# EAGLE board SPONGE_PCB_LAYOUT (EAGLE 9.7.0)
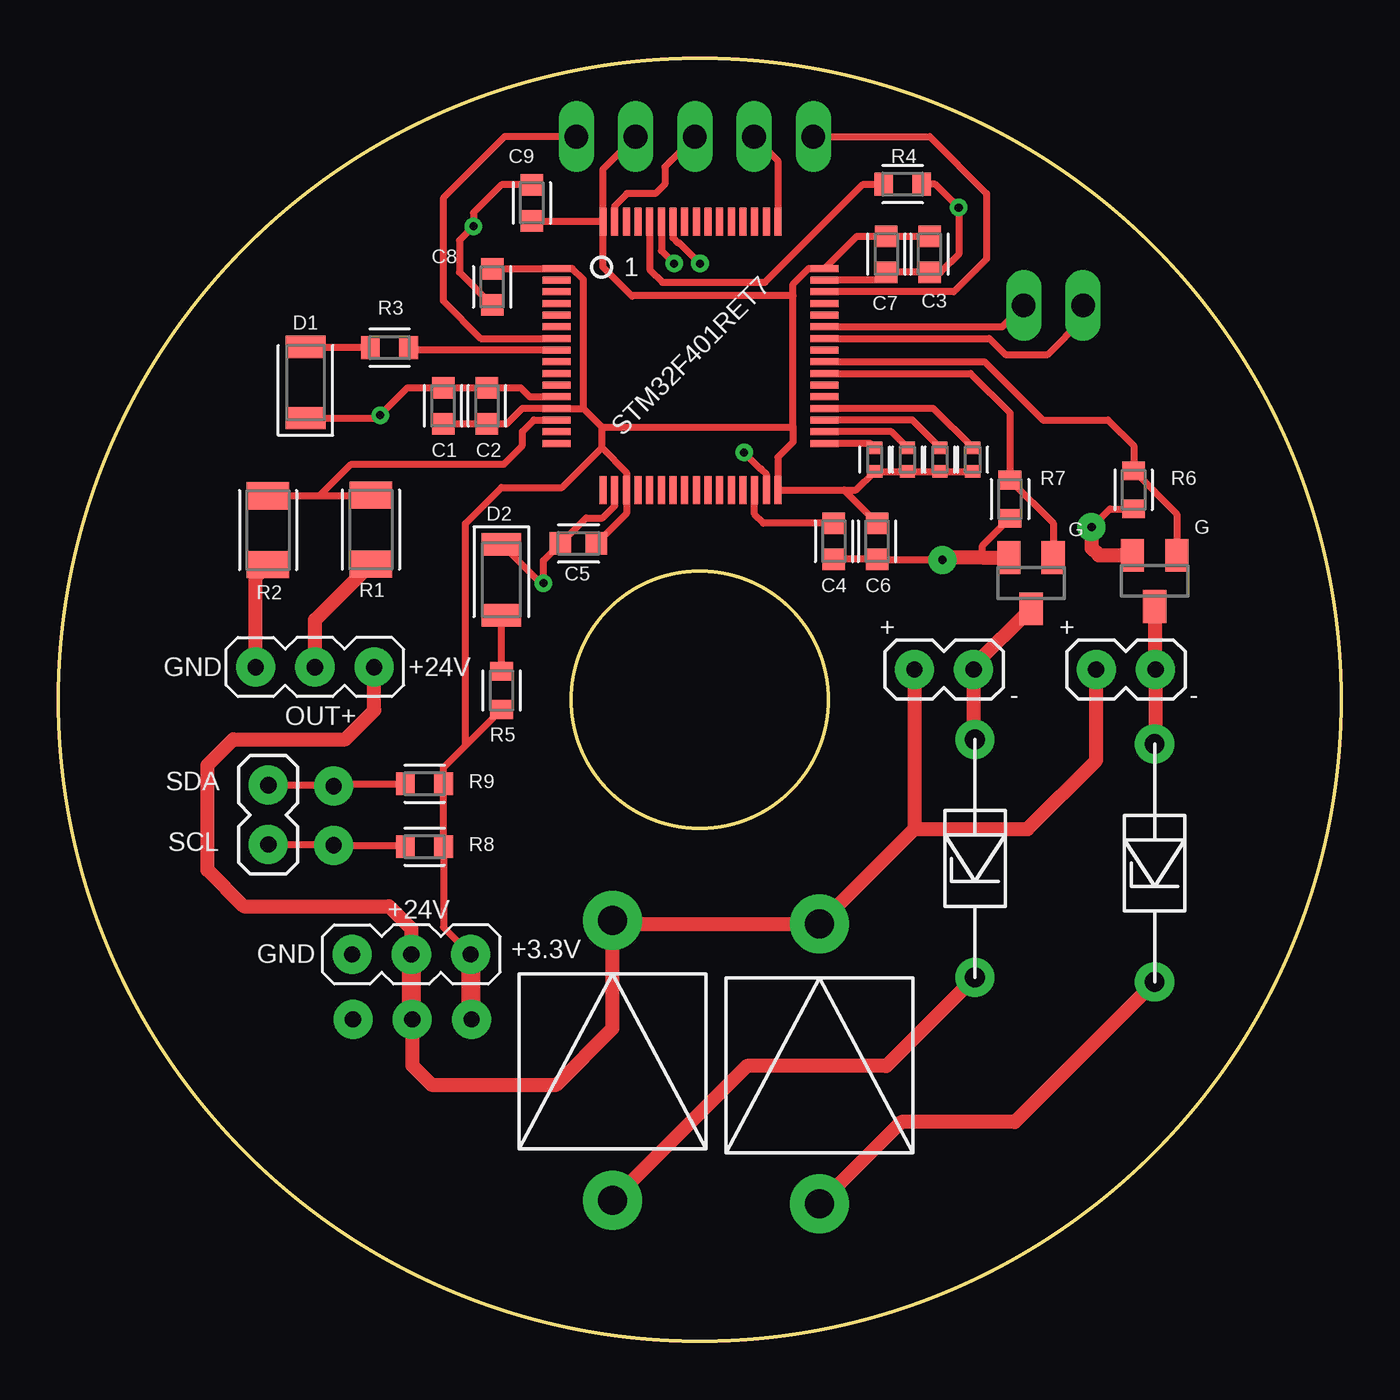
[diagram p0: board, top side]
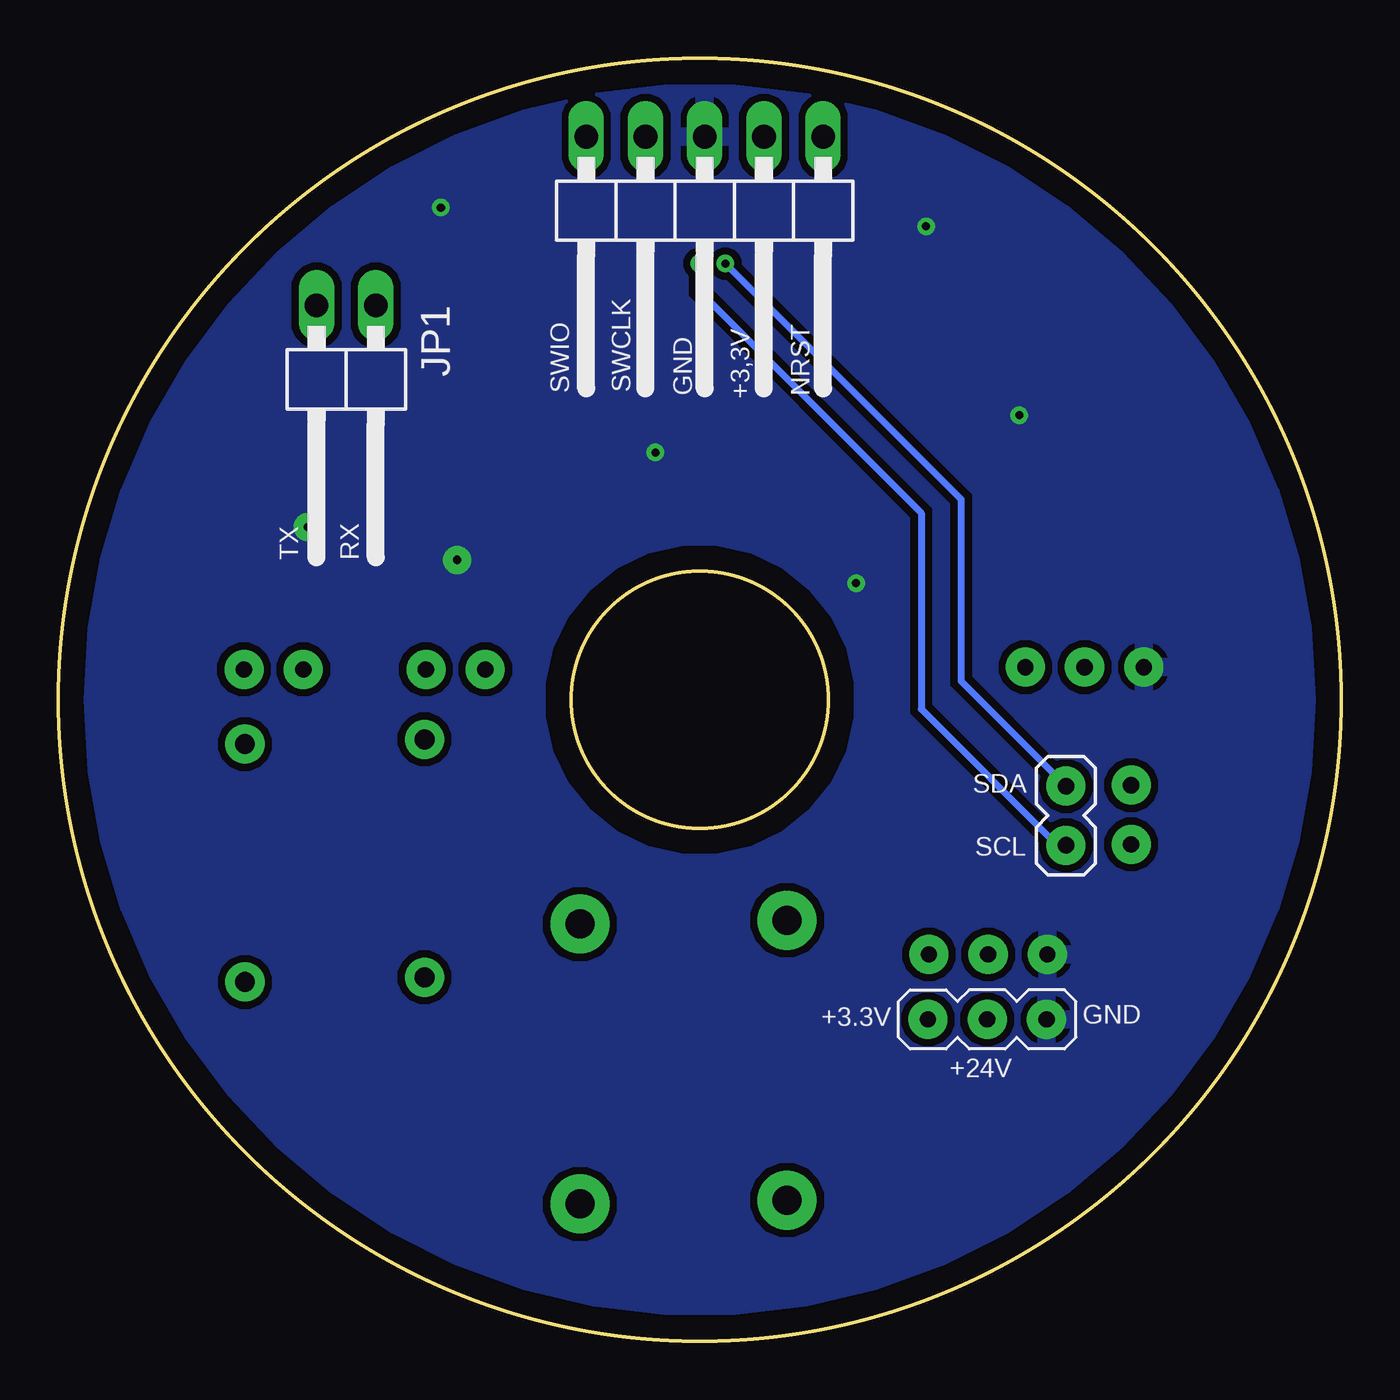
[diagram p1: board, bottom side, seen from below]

Size 55 x 55 mm. Coordinates in mm from the lower left corner, seen from the top.
Outline: circle at 27.5,27.5 radius 5.5
Outline: circle at 27.5,27.5 radius 27.5
Copper layers (1*16): Top / Bottom
Stack-up Default Layer Stack: Top User Defined 0.035mm / Dielectric-1 User Defined 1.5mm / Bottom User Defined 0.035mm
Design rules "default": minimum track width 6mil, minimum drill 0.35mm, track to track 6mil, track to pad 6mil, pad to pad 6mil, via to via 6mil, smd to smd 6mil, copper to edge 40mil, drill to drill 6mil, minimum pad ring 10mil, minimum via ring 8mil, stop-mask expansion 4mil, vias tented up to drill 0mil, thermal gap 10mil

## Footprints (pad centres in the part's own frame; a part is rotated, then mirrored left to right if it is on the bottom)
CAPC1608X85 = smd 0.921 x 0.97: 1 -0.775,0; 2 0.775,0
LEDC3216X75N_FLAT-G = smd 0.962 x 1.712: A 1.525,0; C -1.525,0
1X05/90 = drill 1.016 long: 1 -5.08,-3.81; 2 -2.54,-3.81; 3 0,-3.81; 4 2.54,-3.81; 5 5.08,-3.81
FE3X1 = drill 0.7 pad 1.676: P$1 -2.54,0; P$2 0,0; P$3 2.54,0
1X02/90 = drill 1.016 long: 1 -1.27,-3.81; 2 1.27,-3.81
SOT23 = smd 1 x 1.4: 1 -0.95,-1.1; 2 0.95,-1.1; 3 0,1.1
RESC3216X70 = smd 1.165 x 1.815: 1 -1.475,0; 2 1.475,0
RESC1608X60 = smd 0.799 x 0.974: 1 -0.815,0; 2 0.815,0
RESC1005X40 = smd 0.535 x 0.644: 1 -0.507,0; 2 0.507,0
STM32F401_FOOTPRINT = smd 0.3 x 1.2: BOOT0 -1.75,5.75; PA3 -3.75,-5.75; PA4 -2.25,-5.75; PA5 -1.75,-5.75; PA6 -1.25,-5.75; PA7 -0.75,-5.75; PA14 3.75,5.75; PA15 3.25,5.75; PB0 0.75,-5.75; PB1 1.25,-5.75; PB2 1.75,-5.75; PB3 0.75,5.75; PB4 0.25,5.75; PB5 -0.25,5.75; PB6 -0.75,5.75; PB7 -1.25,5.75; PB8 -2.25,5.75; PB9 -2.75,5.75; PB10 2.25,-5.75; PC4 -0.25,-5.75; PC5 0.25,-5.75; PC10 2.75,5.75; PC11 2.25,5.75; PC12 1.75,5.75; PD2 1.25,5.75; VCAP1 2.75,-5.75; VDD -2.75,-5.75; VDD' 3.75,-5.75; VDD''' -3.75,5.75; VSS -3.25,-5.75; VSS' 3.25,-5.75; VSS''' -3.25,5.75 | smd 1.2 x 0.3: NRST -5.75,0.75; PA0 -5.75,-2.75; PA1 -5.75,-3.25; PA2 -5.75,-3.75; PA8 5.75,0.25; PA9 5.75,0.75; PA10 5.75,1.25; PA11 5.75,1.75; PA12 5.75,2.25; PA13 5.75,2.75; PB12 5.75,-3.75; PB13 5.75,-3.25; PB14 5.75,-2.75; PB15 5.75,-2.25; PC0 -5.75,0.25; PC1 -5.75,-0.25; PC2 -5.75,-0.75; PC3 -5.75,-1.25; PC6 5.75,-1.75; PC7 5.75,-1.25; PC8 5.75,-0.75; PC9 5.75,-0.25; PC13 -5.75,3.25; PC14-OSC32_IN -5.75,2.75; PC15-OSC32_OUT -5.75,2.25; PH0-OSC_IN -5.75,1.75; PH1-OSC_OUT -5.75,1.25; VBAT -5.75,3.75; VDD'' 5.75,3.75; VDDA/VREF+ -5.75,-2.25; VSS'' 5.75,3.25; VSSA/VREF- -5.75,-1.75
IN4005 = drill 1.25 pad 2.54: P$1 0,6; P$2 0,-6
FE2X1 = drill 0.7 pad 1.676: P$1 0,0; P$2 2.54,0
ZENER_1N4757 = drill 0.85 pad 1.676: P$1 0,5.1; P$2 0,-5.1

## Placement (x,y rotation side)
C1  100nF  [CAPC1608X85]  16.5,40.1 270 top
C2  1uF  [CAPC1608X85]  18.38,40.1 270 top
C3  4,7uF  [CAPC1608X85]  37.35,46.6 90 top
C4  4,7uF  [CAPC1608X85]  33.25,34.3 90 top
C5  100nF  [CAPC1608X85]  22.3,34.2 0 top
C6  100nF  [CAPC1608X85]  35.1,34.3 90 top
C7  100nF  [CAPC1608X85]  35.5,46.6 270 top
C8  100nF  [CAPC1608X85]  18.6,45.2 90 top
C9  100nF  [CAPC1608X85]  20.3,48.8 90 top
D1  LED_GREEN  [LEDC3216X75N_FLAT-G]  10.6,41.1 90 top
D2  LED_GREEN  [LEDC3216X75N_FLAT-G]  18.99,32.65 270 top
DEBUG  PINHD-1X5/90  [1X05/90]  27.29,47.83 180 bottom
HALL  FE3X1  [FE3X1]  11,28.9 180 top
JP1  PINHD-1X2/90  [1X02/90]  42.66,40.6 180 bottom
Q1  NMOSFET  [SOT23]  47,32.6 180 top
Q2  NMOSFET  [SOT23]  41.7,32.5 180 top
R1  6k8R  [RESC3216X70]  13.4,34.8 90 top
R2  3k3R  [RESC3216X70]  8.99,34.77 90 top
R3  1kR  [RESC1608X60]  14.2,42.6 180 top
R4  10kR  [RESC1608X60]  36.2,49.6 0 top
R5  1kR  [RESC1608X60]  19,27.9 90 top
R6  10kR  [RESC1608X60]  46.1,36.5 90 top
R7  10kR  [RESC1608X60]  40.8,36.1 90 top
R8  2kR  [RESC1608X60]  15.7,21.2 180 top
R9  2kR  [RESC1608X60]  15.7,23.9 180 top
R10  0R  [RESC1005X40]  39.2,37.8 270 top
R11  0R  [RESC1005X40]  37.8,37.8 270 top
R12  0R  [RESC1005X40]  36.4,37.8 270 top
R13  0R  [RESC1005X40]  35,37.8 270 top
U$1  STM32F401RET7  [STM32F401_FOOTPRINT]  27.1,42.24 0 top
U$2  IN4005  [IN4005]  32.63,11.88 0 top
U$3  IN4005  [IN4005]  23.76,12.04 0 top
U$4  FE3X1  [FE3X1]  15.14,16.58 180 top
U$5  FE3X1  [FE3X1]  15.18,13.8 180 bottom
U$7  FE2X1  [FE2X1]  11.8,23.8 270 bottom
U$8  FE2X1  [FE2X1]  9,21.3 90 top
VENTIL1  FE2X1  [FE2X1]  44.5,28.8 0 top
VENTIL2  FE2X1  [FE2X1]  36.7,28.8 0 top
ZD1  51V  [ZENER_1N4757]  47,20.5 180 top
ZD2  51V  [ZENER_1N4757]  39.3,20.7 180 top

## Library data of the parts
C1-C9 = Capacitor; CATEGORY: Capacitor
D1 D2 = LED; CATEGORY: LED; COLOR: GREEN; DESCRIPTION: CHIP LED FLAT; SUB-CATEGORY: CHIP; TYPE: FLAT_TOP
DEBUG JP1 = Connector; CATEGORY: CONNECTOR; SUB-CATEGORY: PIN-HEADER
HALL U$1-U$5 U$7 U$8 VENTIL1 VENTIL2 ZD1 ZD2 = Haley_Components
Q1 Q2 = Transistor; CATEGORY: Transistor; SUB-CATEGORY: MOSFET; TYPE: N-Channel
R1-R13 = Resistor; CATEGORY: Resistor; SUB-CATEGORY: Fixed

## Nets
+3.3V: C1.2 C2.2 C3.2 C5.2 C6.2 C7.1 C8.2 C9.1 DEBUG.2 R5.1 R8.1 R9.1 R10.2 R11.2 R12.2 R13.2 U$1.VBAT U$1.VDD U$1.VDD' U$1.VDD'' U$1.VDD''' U$1.VDDA/VREF+ U$4.P$1 U$5.P$3
+24V: HALL.P$1 U$2.P$1 U$3.P$1 U$4.P$2 U$5.P$2 VENTIL1.P$1 VENTIL2.P$1
ADC: R1.2 R2.2 U$1.PA0
GND: C1.1 C2.1 C3.1 C4.1 C5.1 C6.1 C7.2 C8.1 C9.2 D1.C D2.C DEBUG.3 HALL.P$3 Q1.2 Q2.2 R2.1 R4.2 R6.1 R7.1 U$1.VSS U$1.VSS' U$1.VSS'' U$1.VSS''' U$1.VSSA/VREF- U$4.P$3 U$5.P$1
ID0: R13.1 U$1.PB12
ID1: R12.1 U$1.PB13
ID2: R11.1 U$1.PB14
ID3: R10.1 U$1.PB15
LED_OUT: R3.1 U$1.PC0
N$1: C4.2 U$1.VCAP1
N$2: R4.1 U$1.BOOT0
N$3: D1.A R3.2
N$5: Q1.3 VENTIL1.P$2 ZD1.P$2
N$6: Q2.3 VENTIL2.P$2 ZD2.P$2
N$7: U$3.P$2 ZD2.P$1
N$8: U$2.P$2 ZD1.P$1
N$9: D2.A R5.2
NRST: DEBUG.1 U$1.NRST
OUT_VENTIL1: Q1.1 R6.2 U$1.PC9
OUT_VENTIL2: Q2.1 R7.2 U$1.PC8
RX: JP1.1 U$1.PA10
SCL: R8.2 U$1.PB6 U$7.P$2 U$8.P$1
SDA: R9.2 U$1.PB7 U$7.P$1 U$8.P$2
SENSOR_OUT+: HALL.P$2 R1.1
SWCLK: DEBUG.4 U$1.PA14
SWIO: DEBUG.5 U$1.PA13
TX: JP1.2 U$1.PA9

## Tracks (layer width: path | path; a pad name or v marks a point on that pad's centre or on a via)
+3.3V
  Top 0.305: 17.46,25.54 16.52,24.6 R9.1 R8.1 16.52,17.74 U$4.P$1 | 17.46,25.54 R5.1 | 17.46,25.54 17.46,35.06 19,36.6 21.6,36.6 23.3,38.3 | C5.2 24.35,35.48 U$1.VDD 24.35,37.25 23.3,38.3 | 23.3,38.3 23.3,39.2 | 22.51,39.99 23.3,39.2 | 22.51,39.99 U$1.VDDA/VREF+ 19.89,39.99 19.23,39.33 C2.2 C1.2 | 22.51,39.99 22.51,45.51 22.03,45.99 U$1.VBAT 21.34,45.98 C8.2 | U$1.VDD''' 23.32,48.02 C9.1 | U$1.VDD''' 23.35,50.24 DEBUG.2 | 33.69,36.49 U$1.VDD' 30.85,37.9 31.5,38.55 31.5,39.2 | 33.69,36.49 C6.2 | 33.69,36.49 34.2,36.49 R13.2 R12.2 R11.2 R10.2 | 31.5,39.2 31.5,44.82 | 31.5,44.82 31.5,45.32 32.17,45.99 U$1.VDD'' 34.23,47.38 C7.1 C3.2 | 31.5,44.82 24.62,44.82 24.6,44.8 23.35,46.05 U$1.VDD''' | 23.3,39.2 31.5,39.2
  Top 0.813: U$4.P$1 17.68,13.84 U$5.P$3
+24V
  Top 0.61: 36.7,21.95 U$2.P$1 23.92,17.88 U$3.P$1 23.76,13.41 21.35,11 16,11 15.18,11.82 U$5.P$2 | VENTIL2.P$1 36.7,21.95 | 36.7,21.95 41.55,21.95 44.5,24.9 VENTIL1.P$1 | HALL.P$1 13.54,27.04 12.3,25.8 7.5,25.8 6.4,24.7 6.4,20.2 7.95,18.65 14.17,18.65 15.14,17.69 U$4.P$2
  Top 0.813: U$4.P$2 15.14,13.84 U$5.P$2
ADC
  Top 0.305: R2.2 11.2,36.24 | 11.2,36.24 13.37,36.24 R1.2 | 11.2,36.24 12.55,37.6 19.1,37.6 19.9,38.4 19.9,39 20.39,39.49 U$1.PA0
GND  (via drill 0.35, 0.35 pad 1.2)
  Top 0.305: DEBUG.3 26,50.35 26,49.6 25.6,49.2 24.38,49.2 23.85,48.67 U$1.VSS''' | C9.2 19,49.58 17.8,48.38 v17.8,47.8 17.2,47.2 17.2,45.83 C8.1 | D1.C 13.68,39.58 v13.8,39.7 14.97,40.88 C1.1 C2.1 19.82,40.88 20.21,40.49 U$1.VSSA/VREF- | D2.C 20.66,32.5 v20.8,32.5 20.8,33.48 C5.1 22.62,35.3 23.34,35.3 23.85,35.81 U$1.VSS | v29.4,38.1 30.11,37.39 30.13,37.39 30.35,37.17 U$1.VSS' | C4.1 C6.1 35.12,33.5 v37.9,33.5 38,33.6 | R7.1 39.6,34.09 39.6,33.6 | v44.3,34.9 45.09,35.69 R6.1 | R4.2 37.6,49.6 v38.6,48.6 38.6,46.6 37.83,45.83 C3.1 C7.2 35.16,45.49 U$1.VSS''
  Top 0.61: HALL.P$3 8.46,32.76 R2.1 | 38,33.6 39.6,33.6 Q2.2 | v44.3,34.9 44.3,34 44.6,33.7 Q1.2
  pour Bottom (isolate 0.305): 27,55 25.2,54.9 23.4,54.7 21.8,54.4 20.2,54 19.5,53.8 18.3,53.4 16.7,52.8 15.2,52.1 13.7,51.3 12,50.2 10.6,49.2 8.6,47.5 6.9,45.7 5.6,44.1 4.4,42.4 3.1,40.2 2,37.8 1,34.9 0.6,33.2 0.2,30.9 0.2,26.56 0.58,22.03 0.9,20.5 1.4,18.8 1.9,17.4 2.5,16 3.3,14.4 4.32,12.82 6.7,9.79 10,6.3 12,4.8 13.7,3.7 15.8,2.6 18.2,1.6 20.9,0.8 22.2,0.5 23.3,0.3 24,0.2 26.2,0 28.2,0 29.8,0.1 31.5,0.3 32.8,0.5 33.8,0.7 37.6,1.9 39,2.5 41,3.5 42.3,4.3 44.3,5.7 45.3,6.5 46.4,7.5 47.9,9 48.9,10.2 50.4,12.2 51,13.2 52.1,15.1 52.7,16.5 53.7,19.1 54.3,21.3 54.8,24 55,26.2 55,28 54.9,29.9 54.6,32.2 54.2,34.1 53.6,36.2 53.1,37.6 52.6,38.7 52,40 51.3,41.3 50.5,42.6 49.5,44 48.8,44.9 48.2,45.6 46.6,47.3 46.1,47.75 44,49.5 43.3,50 42.3,50.7 40.6,51.7 39,52.5 37.3,53.2 35.5,53.8 34.1,54.2 32.8,54.5 31.5,54.7 30.8,54.8 29.7,54.9 27.9,55
ID0
  Top 0.305: R13.1 34.82,38.49 U$1.PB12
ID1
  Top 0.305: U$1.PB13 35.72,38.99 R12.1
ID2
  Top 0.305: U$1.PB14 36.62,39.49 R11.1
ID3
  Top 0.305: U$1.PB15 37.52,39.99 R10.1
LED_OUT
  Top 0.305: U$1.PC0 15.12,42.49 R3.1
N$1
  Top 0.305: C4.2 30.23,35.08 29.85,35.45 U$1.VCAP1
N$2
  Top 0.305: U$1.BOOT0 25.35,45.95 25.9,45.4 30.3,45.4 34.5,49.6 R4.1
N$3
  Top 0.305: R3.2 10.62,42.6 D1.A
N$5
  Top 0.305: 47,28.84 VENTIL1.P$2 | 47.04,25.64 ZD1.P$2
  Top 0.61: Q1.3 47,28.84 | VENTIL1.P$2 47.04,25.64
N$6
  Top 0.305: 39.24,28.94 VENTIL2.P$2 | 39.24,25.86 ZD2.P$2
  Top 0.61: Q2.3 39.24,28.94 | VENTIL2.P$2 39.24,25.86
N$7
  Top 0.61: ZD2.P$1 35.5,11.8 29.52,11.8 U$3.P$2
N$8
  Top 0.61: ZD1.P$1 41,9.4 36.15,9.4 U$2.P$2
N$9
  Top 0.305: R5.2 D2.A
NRST
  Top 0.305: DEBUG.1 19.14,51.64 16.5,49 16.5,44.6 18.11,42.99 U$1.NRST
OUT_VENTIL1
  Top 0.305: U$1.PC9 39.71,41.99 42.2,39.5 45,39.5 46.1,38.4 R6.2 47.95,35.47 Q1.1
OUT_VENTIL2
  Top 0.305: U$1.PC8 39.11,41.49 40.8,39.8 R7.2 42.65,35.06 Q2.1
RX
  Top 0.305: U$1.PA10 40.47,43.49 JP1.1
SCL  (via drill 0.35 pad 0.55)
  Top 0.305: U$8.P$1 11.76,21.3 U$7.P$2 14.82,21.26 R8.2 | v27.51,46.2 26.62,47.09 26.57,47.09 26.35,47.31 U$1.PB6
  Bottom 0.305: U$7.P$2 12.16,21.26 18,27.1 18,35.5 27.51,45.01 v27.51,46.2
SDA  (via drill 0.35)
  Top 0.305: U$8.P$2 11.76,23.84 U$7.P$1 11.9,23.9 R9.2 | U$1.PB7 25.85,46.75 v26.4,46.2
  Bottom 0.305: v26.4,46.2 16.3,36.1 16.3,28.3 U$7.P$1
SENSOR_OUT+
  Top 0.61: HALL.P$2 11,30.93 R1.1
SWCLK
  Top 0.305: DEBUG.4 30.85,50.62 U$1.PA14
SWIO
  Top 0.305: DEBUG.5 37.36,51.64 39.8,49.2 39.8,46.4 38.39,44.99 U$1.PA13
TX
  Top 0.305: U$1.PA9 39.91,42.99 40.6,42.3 42.42,42.3 43.93,43.81 JP1.2

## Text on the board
tPlace: G | G
bPlace: SWIO
tNames: C9 | R4 | C8 | C7 | C3 | R3 | C1 | C2 | R7 | R6 | C5 | C4 | C6 | R2 | R1 | + | + | GND | +24V | - | - | OUT+ | R5 | SDA | R9 | SCL | R8 | +24V | GND | +3.3V
bNames: SWCLK | NRST | +3,3V | GND | RX | TX | SDA | SCL | GND | +3.3V | +24V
